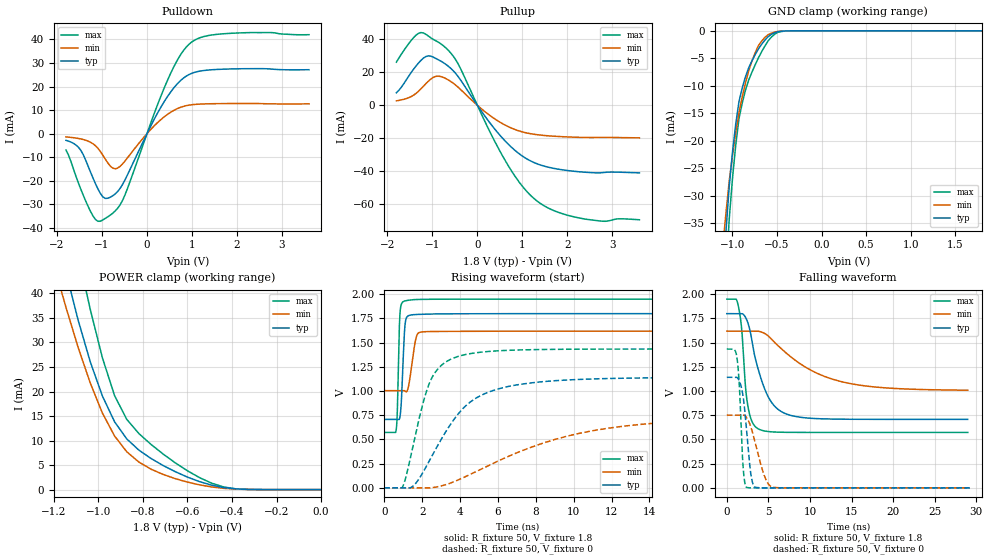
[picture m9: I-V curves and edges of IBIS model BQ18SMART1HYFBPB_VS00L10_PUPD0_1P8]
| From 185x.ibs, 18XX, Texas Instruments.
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|   Model Cell BQ18SMART1HYFBPB_VS00L10_PUPD0_1P8
|BQ18SMART1HYFBPB_VS00L10_PUPD0_1P8
[Model]   BQ18SMART1HYFBPB_VS00L10_PUPD0_1P8
Model_type   I/O
Polarity   Non-Inverting
Enable   Active-Low
Vinl =  0.63
Vinh =  1.17
Cref =  15pF
Rref =  100.0000M
Vref =  0V
Vmeas =  0.9
C_comp   0.9029199p   0.7983694p   1.014934p
[Model Spec]
Vinl   0.63   0.567   0.6825
Vinh   1.17   1.053   1.2675
[Temperature Range]   25   125   -40
[Voltage Range]   1.8   1.62   1.95
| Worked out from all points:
|   slope of the pulldown table from 0 to 0.27 V, typ, clamps not added: 27.2 ohm
|   slope of the pullup table from 0 to 0.27 V, typ, clamps not added: 26 ohm
|   GND clamp passes 1 mA (typ) near -0.59 V on its own axis
|   POWER clamp passes 1 mA (typ) near -0.50 V on its own axis
|   rising waveform, R_fixture 50, V_fixture 1.8: 20-80 % time 147ps typ, 270ps min, 101ps max; typ from 0.707 V to 1.8 V
|   rising waveform, R_fixture 50, V_fixture 0: 20-80 % time 2.5ns typ, 6.49ns min, 1.19ns max; typ from 0 V to 1.14 V
|   falling waveform, R_fixture 50, V_fixture 1.8: 20-80 % time 2.17ns typ, 6.59ns min, 777ps max; typ from 1.8 V to 0.708 V
|   falling waveform, R_fixture 50, V_fixture 0: 20-80 % time 757ps typ, 1.42ns min, 464ps max; typ from 1.14 V to 0 V
| Nom Voltages:
|   BIASFET=1.8, VBBNW=1.1, VDD=1.1, VDDS=1.8, VSS=0, VSSS=0
| Min Voltages:
|   BIASFET=1.62, VBBNW=0.99, VDD=0.99, VDDS=1.62, VSS=0, VSSS=0
| Max Voltages:
|   BIASFET=1.95, VBBNW=1.21, VDD=1.21, VDDS=1.95, VSS=0, VSSS=0
[POWER_clamp]
|   voltage   I(typ)   I(min)   I(max)
-1.8V     196.8mA    157.5mA    250.4mA
-1.164V   48mA       40.06mA    64.23mA
-1.127V   41.11mA    34.43mA    55.95mA
-1.109V   37.83mA    31.72mA    51.94mA
-1.055V   28.88mA    24.15mA    40.47mA
-981.8mV  19.06mA    15.6mA     26.85mA
-927.3mV  13.83mA    10.93mA    19.15mA
-872.7mV  10.34mA    7.72mA     14.33mA
-763.6mV  6.344mA    4.165mA    9.211mA
-600mV    2.546mA    1.527mA    3.832mA
-436.4mV  402.5uA    253uA      527.5uA
0V        291.8pA    1.073nA    4.224nA
[Pulldown]
|   voltage   I(typ)   I(min)   I(max)
-1.8V     -2.835mA   -1.376mA   -6.938mA
-1.473V   -6.994mA   -2.229mA   -23.44mA
-1.2V     -18.79mA   -4.282mA   -34.89mA
-1.036V   -25.33mA   -7.531mA   -37.14mA
-872.7mV  -27.39mA   -12.36mA   -35.28mA
-654.5mV  -24.59mA   -14.63mA   -31.68mA
-490.9mV  -19.69mA   -11.65mA   -26.08mA
381.8mV   13.54mA    7.117mA    19.32mA
654.5mV   20.72mA    10.44mA    30.48mA
927.3mV   25mA       12.07mA    37.79mA
1.636V    27.3mA     12.74mA    42.26mA
3.6V      27.12mA    12.64mA    41.97mA
[Pullup]
|   voltage   I(typ)   I(min)   I(max)
-1.8V     7.614mA    2.74mA     26.22mA
-1.527V   17.69mA    4.626mA    37.43mA
-1.309V   25.69mA    8.541mA    43.72mA
-1.036V   29.87mA    15.94mA    41.05mA
-818.2mV  26.95mA    17.52mA    37.49mA
-490.9mV  19.61mA    12.45mA    28.08mA
545.5mV   -19.54mA   -10.94mA   -30.03mA
927.3mV   -29.38mA   -15.56mA   -46.58mA
1.255V    -34.7mA    -17.56mA   -56.51mA
1.691V    -38.25mA   -18.74mA   -63.85mA
2.291V    -40.42mA   -19.45mA   -68.55mA
3.6V      -41.01mA   -19.75mA   -69.5mA
[GND_clamp]
|   voltage   I(typ)   I(min)   I(max)
-1.8V     -274mA     -200.4mA   -365.5mA
-1.109V   -45.37mA   -39.32mA   -55.85mA
-1.073V   -36.45mA   -33.1mA    -44.39mA
-1.036V   -28.3mA    -27.35mA   -34.22mA
-1V       -22.14mA   -22.69mA   -26.92mA
-927.3mV  -12.91mA   -14.91mA   -16.03mA
-854.5mV  -8.387mA   -9.532mA   -10.83mA
-781.8mV  -5.484mA   -5.512mA   -7.535mA
-709.1mV  -3.298mA   -2.71mA    -4.931mA
-600mV    -1.058mA   -705.2uA   -1.831mA
-381.8mV  -13.32uA   -12.31uA   -19.39uA
1.8V      291.8pA    820.3nA    4.087nA
[Ramp]
| variable   typ   min   max
dV/dt_f 0.65751256/2.1762577n 0.37052149/6.6939513n 0.82843094/0.77956186n
dV/dt_r 0.69719994/2.5124826n 0.45743512/6.7022415n 0.87612418/1.1983027n
R_load = 50
[Rising Waveform]
R_fixture = 50
V_fixture = 1.8
V_fixture_min = 1.62
V_fixture_max = 1.95
|   time   V(typ)   V(min)   V(max)
0s        707.2mV    1.005V     572.6mV
626.4ps   707.2mV    1.005V     593.3mV
689.9ps   707.2mV    1.005V     790.6mV
828.6ps   732.9mV    1.005V     1.795V
904.5ps   897.4mV    1.005V     1.898V
1.104ns   1.696V     998.7mV    1.932V
1.286ns   1.779V     1.054V     1.939V
1.687ns   1.791V     1.555V     1.946V
1.99ns    1.794V     1.611V     1.948V
28.98ns   1.8V       1.62V      1.95V
[Rising Waveform]
R_fixture = 50
V_fixture = 0
V_fixture_min = 0
V_fixture_max = 0
|   time   V(typ)   V(min)   V(max)
0s        0V         0V         0V
939.8ps   0V         0V         0V
1.605ns   34.25mV    0V         512.8mV
2.44ns    300.9mV    0V         1.107V
3.097ns   531.6mV    23.99mV    1.279V
4.147ns   817.8mV    103.1mV    1.371V
5.191ns   963.1mV    201.3mV    1.404V
6.686ns   1.053V     336.5mV    1.422V
12.26ns   1.132V     628.1mV    1.434V
29.23ns   1.143V     743.4mV    1.434V
[Falling Waveform]
R_fixture = 50
V_fixture = 1.8
V_fixture_min = 1.62
V_fixture_max = 1.95
|   time   V(typ)   V(min)   V(max)
0s        1.8V       1.619V     1.95V
1.329ns   1.8V       1.619V     1.9V
1.784ns   1.8V       1.619V     1.645V
2.216ns   1.768V     1.619V     1.077V
2.516ns   1.71V      1.619V     854mV
3.782ns   1.223V     1.618V     609.5mV
5.434ns   876.9mV    1.531V     578.3mV
7.834ns   745.6mV    1.344V     573.1mV
15.01ns   708.5mV    1.075V     572.6mV
28.98ns   707.6mV    1.009V     572.6mV
[Falling Waveform]
R_fixture = 50
V_fixture = 0
V_fixture_min = 0
V_fixture_max = 0
|   time   V(typ)   V(min)   V(max)
0s        1.142V     751.5mV    1.434V
1.238ns   1.14V      751.5mV    1.334V
1.506ns   1.104V     751.5mV    1.06V
1.962ns   943.6mV    751.5mV    214.6mV
2.35ns    621.4mV    729.6mV    6.135mV
2.829ns   183.2mV    645.8mV    0V
3.2ns     28.9mV     537.9mV    0V
4.529ns   0V         122.9mV    0V
5.461ns   0V         8.557mV    0V
29.23ns   0V         0V         0V
